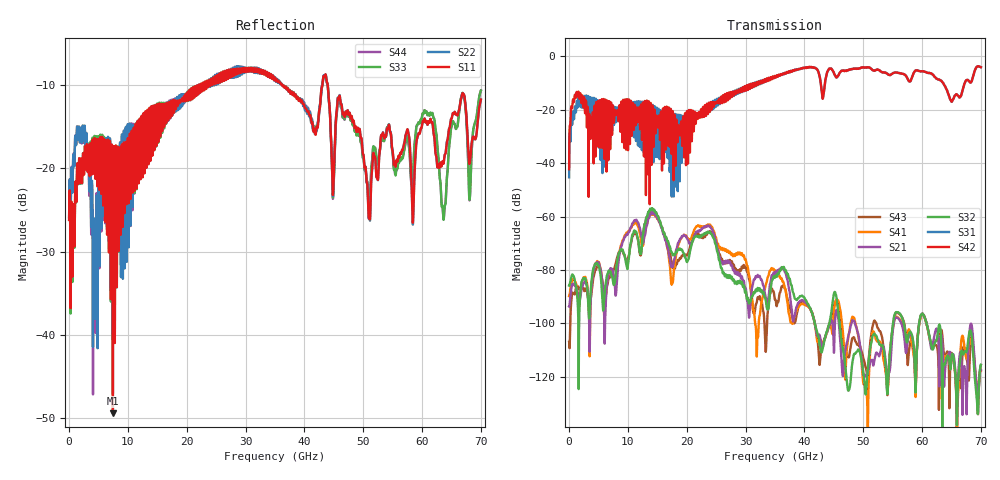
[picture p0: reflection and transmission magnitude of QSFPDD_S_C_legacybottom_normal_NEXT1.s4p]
! AWR Design Environment (8415) Thu Dec 20 15:16:03 2018
! Document = 'CHANNEL TEST'
! nPorts: 4, nXvals: 7001
# HZ S DB R 50
!Freq DBS11 AngS11 DBS12 AngS12 DBS13 AngS13 DBS14 AngS14
!	DBS21 AngS21 DBS22 AngS22 DBS23 AngS23 DBS24 AngS24
!	DBS31 AngS31 DBS32 AngS32 DBS33 AngS33 DBS34 AngS34
!	DBS41 AngS41 DBS42 AngS42 DBS43 AngS43 DBS44 AngS44
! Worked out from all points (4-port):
!   7000 points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, 10 MHz to 70 GHz, reference 50 ohm
!   strongest paths, dB at 10 MHz, 17.51 GHz, 35.01 GHz, 52.51 GHz, 70 GHz:
!     S42: -42.2, -24.0, -7.5, -5.0, -4.0
!     S31: -45.3, -28.7, -7.5, -5.0, -4.0
!     S32: -85.9, -73.6, -82.8, -106.3, -115.5
!     S21: -93.7, -78.6, -81.3, -111.4, -117.5
!     S41: -89.8, -85.1, -80.3, -106.5, -117.7
!     S43: -106.9, -77.4, -91.1, -101.8, -115.6
!   lowest |S11| = -49.4 dB at 7.45 GHz (marker M1), VSWR 1.01, Z = 50.3 + j0.0931 ohm
!   |S11| at or under -10 dB: start of sweep to 22.1 GHz; 36.25 GHz to 43.06 GHz (6.813 GHz wide, 17.2 % of centre); 43.96 GHz to end of sweep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
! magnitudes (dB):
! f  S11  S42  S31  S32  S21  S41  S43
! 10 MHz  -26.2  -42.2  -45.3  -85.9  -93.7  -89.8  -106.9
! 1.3 GHz  -21.9  -13.3  -16.9  -87.9  -87.2  -86.5  -86.3
! 7.45 GHz  -49.4  -18.4  -18.5  -84.0  -80.4  -81.4  -80.6
! 14.08 GHz  -14.4  -25.8  -29.9  -56.8  -58.3  -58.6  -57.0
! 17.86 GHz  -13.1  -23.8  -26.7  -74.2  -76.1  -79.2  -79.0
! 23.74 GHz  -9.7  -17.4  -18.5  -66.0  -63.6  -63.2  -66.0
! 70 GHz  -11.8  -4.0  -4.0  -115.5  -117.5  -117.7  -115.6
